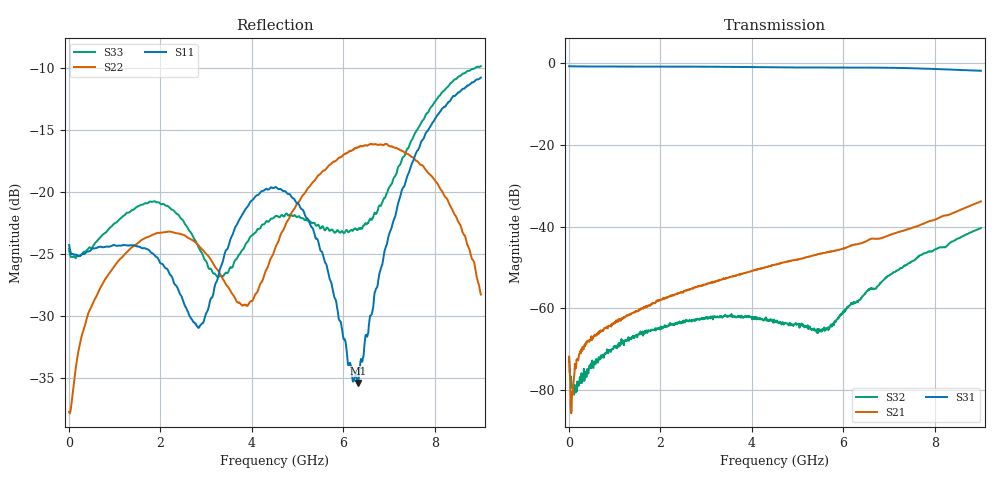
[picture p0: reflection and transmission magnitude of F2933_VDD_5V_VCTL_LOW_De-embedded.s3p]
! Integrated Device Technology
! Corporate Headquarters
! 6024 Silver Creek Valley Road
! San Jose, CA 95138  USA
! Phone:  1-408-284-8200
! Toll Free:  1-800-223-1366
! Webpage:  http://www.idt.com/
! Timing and RF Division
! 515 Groton Road, Suite 102
! Westford, MA 01886-6024
! Device:  F2933
! Description: 50 Ohm SP2T RF Switch
! Frequency:  50 MHz to 8 GHz
! Package:  4 mm x 4 mm QFN Plastic Package: 16-pin
! Ports:  3 RF, 2 DC
!  Pin  1  = VDD
!  Pin  2  = VCTL
!  Pin  3  = RFC  = Port 3
!  Pin  4  = GND
!  Pin  5  = GND
!  Pin  6  = GND
!  Pin  7  = GND
!  Pin  8  = GND
!  Pin  9  = RF2	= Port 2
!  Pin  10  = GND
!  Pin  11  = GND
!  Pin  12  = RF1	= Port 1
!  Pin  13  = GND
!  Pin  14  = GND
!  Pin  15  = GND
!  Pin  16  = GND
!  EP  = GND
! State:  RF1 selected
! EVKIT Voltages:		VDD  = +5.0 V
!  VCTL = 0 V (Logic LOW)
! Data:  The device was measured on the F2932 EVKit
!  using a calibrated network analyzer with the following
!  EVKIT modifications:
!  R1 = 5.1k ohm
!  C4 = 10 pF
!  These modifications improve the high frequency performance since
!  the standard EVKIT layout has some RF coupling between RFC (pin 3)
!  and VCTL (pin 2).
!  The evaluation board was de-embedded using Automatic Fixture Removal (AFR).
!  The reference plane is the edge of the package pin.
! Misc:
! Date Measured:  2018-5-16
! Date:  2018-5-16
! Note:
!  Integrated Device Technology supplies this data as a sample
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# hz S db R 50
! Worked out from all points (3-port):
!   1000 points, 10 MHz to 9 GHz, reference 50 ohm
!   strongest paths, dB at 10 MHz, 2.26 GHz, 4.509 GHz, 6.759 GHz, 9 GHz:
!     S31: -0.7, -0.8, -1.0, -1.0, -1.8
!     S21: -71.8, -56.8, -49.3, -42.9, -33.8
!     S32: -72.0, -64.0, -63.3, -54.4, -40.3
!   lowest |S11| = -35.4 dB at 6.309 GHz (marker M1), VSWR 1.03, Z = 48.6 + j0.874 ohm
!   |S11| at or under -10 dB: start of sweep to end of sweep
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1e7  -24.26 -2.2  -71.54 -7.1  -0.68 -0.4
     -71.79 -5.3  -37.71 -0.5  -71.54 -19.0
     -0.68 -0.3  -72.04 -16.6  -24.57 -1.8
1.35986e8  -25.04 5.1  -74.44 65.6  -0.73 -2.7
           -73.57 53.8  -34.73 37.0  -80.77 -134.4
           -0.73 -2.7  -79.61 -136.2  -25.24 2.3
1.062883e9  -24.33 30.1  -62.83 70.5  -0.78 -19.5
            -63.12 70.6  -25.65 63.5  -68.73 118.4
            -0.78 -19.5  -69.08 112.2  -22.36 10.7
2.844685e9  -30.92 -31.9  -54.60 85.1  -0.80 -52.2
            -54.57 86.0  -24.34 76.7  -62.55 62.6
            -0.80 -52.2  -62.62 63.6  -24.51 -41.1
3.852573e9  -21.42 -111.5  -51.36 87.9  -0.89 -71.4
            -51.36 87.1  -29.06 34.9  -62.10 29.7
            -0.89 -71.4  -61.91 29.2  -24.29 -138.1
4.5095e9  -19.61 -123.9  -49.33 87.6  -0.97 -83.7
          -49.28 87.9  -24.49 -10.7  -63.36 -2.1
          -0.97 -83.7  -63.25 -1.6  -21.95 -157.3
5.49039e9  -24.63 -141.3  -46.59 88.4  -1.00 -101.9
           -46.57 89.1  -18.54 -18.7  -65.75 -74.2
           -1.00 -101.9  -65.22 -77.8  -22.93 -155.7
6.309299e9  -35.39 148.0  -44.25 91.3  -1.00 -117.8
            -44.29 91.1  -16.41 -15.5  -58.11 -119.4
            -1.00 -117.8  -58.32 -120.4  -23.06 -153.6
7.56016e9  -17.07 98.6  -40.02 93.5  -1.21 -143.1
           -40.00 93.4  -17.37 -8.7  -48.09 -160.5
           -1.21 -143.1  -48.12 -160.8  -15.25 154.2
9e9  -10.76 71.3  -33.80 88.8  -1.79 -171.2
     -33.78 88.9  -28.25 -10.8  -40.26 172.3
     -1.79 -171.3  -40.32 172.2  -9.84 124.2
